(* Logix 5000 AddOnInstructionDefinition export V430_Copy_Input_Large_101; software revision 33.01 *)

TYPE INPUT_Large_101 :
STRUCT
   User_Tag_Echo : DINT;
   Command : V430_100_101_Command_Echo;
   Output_Cmd : V430_100_101_Ext_Output_Echo;
   Ext_Input_Status : V430_100_101_Ext_Input_Status;
   Ext_Output_Status : V430_100_101_Ext_Output_Status;
   Device_Status : V430_101_Device_Status;
   Read_Cycle_Sequence_Counter : DINT;
   Trigger_Counter : DINT;
   Decode_Match_Counter : DINT;
   Mismatch_Counter : DINT;
   NoRead_Counter : DINT;
   Decode_Data : V430_Large_128_Char_Str;
END_STRUCT
END_TYPE

TYPE OUTPUT_198 :
STRUCT
   UserTag : DINT;
   Commands : V430_198_Commands;
   Ext_Outputs : V430_198_Ext_Output;
END_STRUCT
END_TYPE

TYPE V430_100_101_Command_Echo :
STRUCT
   Trigger_Echo : BOOL;
   New_Master_Echo : BOOL;
   Reserved01 : BOOL;
   Reserved02 : BOOL;
   Reserved03 : BOOL;
   Reserved04 : BOOL;
   Reserved05 : BOOL;
   Reserved06 : BOOL;
   Disable_Scanning_Echo : BOOL;
   Reserved07 : BOOL;
   Reserved08 : BOOL;
   Reserved09 : BOOL;
   Reserved10 : BOOL;
   Reserved11 : BOOL;
   Reserved12 : BOOL;
   Reserved13 : BOOL;
   Clear_Read_Cycle_Report_and_Counts_Echo : BOOL;
   Unlatch_Outputs_Echo : BOOL;
   Reserved14 : BOOL;
   Reserved15 : BOOL;
   Reserved16 : BOOL;
   Reserved17 : BOOL;
   Reserved18 : BOOL;
   Reserved19 : BOOL;
   Reserved : SINT;
END_STRUCT
END_TYPE

TYPE V430_100_101_Ext_Input_Status :
STRUCT
   Trigger : BOOL;
   New_Master : BOOL;
   Reserved01 : BOOL;
   Reserved02 : BOOL;
   Reserved03 : BOOL;
   Reserved04 : BOOL;
   Reserved05 : BOOL;
   Reserved06 : BOOL;
   Reserved07 : SINT;
   Reserved08 : INT;
END_STRUCT
END_TYPE

TYPE V430_100_101_Ext_Output_Echo :
STRUCT
   Output1_Echo : BOOL;
   Output2_Echo : BOOL;
   Output3_Echo : BOOL;
   Reserved01 : BOOL;
   Reserved02 : BOOL;
   Reserved03 : BOOL;
   Reserved04 : BOOL;
   Reserved05 : BOOL;
   Reserved06 : INT;
END_STRUCT
END_TYPE

TYPE V430_100_101_Ext_Output_Status :
STRUCT
   Output1 : BOOL;
   Output2 : BOOL;
   Output3 : BOOL;
   Reserved01 : BOOL;
   Reserved02 : BOOL;
   Reserved03 : BOOL;
   Reserved04 : BOOL;
   Reserved05 : BOOL;
   Reserved06 : INT;
END_STRUCT
END_TYPE

TYPE V430_101_Device_Status :
STRUCT
   Reserved00 : BOOL;
   New_Master_Requested : BOOL;
   Reserved01 : BOOL;
   Reserved02 : BOOL;
   Reserved03 : BOOL;
   Reserved04 : BOOL;
   Reserved05 : BOOL;
   Reserved06 : BOOL;
   Scanning_Disabled : BOOL;
   Reserved07 : BOOL;
   Reserved08 : BOOL;
   Reserved09 : BOOL;
   Reserved10 : BOOL;
   Reserved11 : BOOL;
   Reserved12 : BOOL;
   Reserved13 : BOOL;
   In_Read_Cycle : BOOL;
   Actively_Scanning : BOOL;
   Reserved14 : BOOL;
   Reserved15 : BOOL;
   Reserved16 : BOOL;
   Reserved17 : BOOL;
   Reserved18 : BOOL;
   Reserved19 : BOOL;
   Reserved : SINT;
END_STRUCT
END_TYPE

TYPE V430_198_Commands :
STRUCT
   Trigger : BOOL;
   New_Master : BOOL;
   Reserved01 : BOOL;
   Reserved02 : BOOL;
   Reserved03 : BOOL;
   Reserved04 : BOOL;
   Reserved05 : BOOL;
   Reserved06 : BOOL;
   Disable_Scanning : BOOL;
   Reserved07 : BOOL;
   Reserved08 : BOOL;
   Reserved09 : BOOL;
   Reserved10 : BOOL;
   Reserved11 : BOOL;
   Reserved12 : BOOL;
   Reserved13 : BOOL;
   Clear_Read_Cycle_Report_and_Counters : BOOL;
   Unlatch_Outputs : BOOL;
   Reserved14 : BOOL;
   Reserved15 : BOOL;
   Reserved16 : BOOL;
   Reserved17 : BOOL;
   Reserved18 : BOOL;
   Reserved19 : BOOL;
   Reserved : SINT;
END_STRUCT
END_TYPE

TYPE V430_198_Ext_Output :
STRUCT
   Output1 : BOOL;
   Output2 : BOOL;
   Output3 : BOOL;
   Reserved01 : BOOL;
   Reserved02 : BOOL;
   Reserved03 : BOOL;
   Reserved04 : BOOL;
   Reserved05 : BOOL;
   Reserved06 : INT;
END_STRUCT
END_TYPE

TYPE V430_Large_128_Char_Str :   // string type
STRUCT
   LEN : DINT;
   DATA : SINT[128];
END_STRUCT
END_TYPE

ADD_ON_INSTRUCTION V430_Copy_Input_Large_101   (* revision 1.0, vendor OMRON *)
// Copies Omron V430-F reader EtherNet/IP input and output assemblies to local tags.
// Requires use of Input Large (101) and Output (198) assemblies.
VAR_IN_OUT
   Assembly_Input : INPUT_Large_101; {required}   // User MicroHAWK Input Assembly
   Assembly_Output : OUTPUT_198; {required}   // User MicroHAWK Output Assembly
   Connection_Input : SINT[176]; {required}   // EIP Input Connection
   Connection_Output : SINT[12]; {required}   // EIP Output Connection
END_VAR

ROUTINE Logic   (* ladder *)
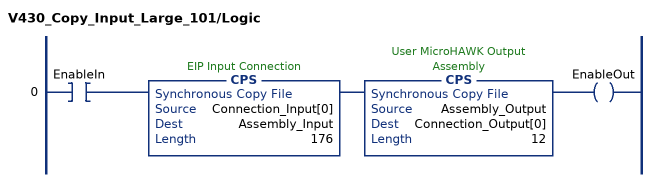
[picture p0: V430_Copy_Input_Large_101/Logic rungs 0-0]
   0: XIC(EnableIn)CPS(Connection_Input[0],Assembly_Input,176)CPS(Assembly_Output,Connection_Output[0],12)OTE(EnableOut);
END_ROUTINE
END_ADD_ON_INSTRUCTION
